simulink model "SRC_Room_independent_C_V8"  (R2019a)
settings: Solver=VariableStepAuto  StartTime=0.0  StopTime=tend  RelTol=1e-6
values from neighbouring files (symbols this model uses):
  initial_switch = zeros(10,1)    [Main_delayV8.m]
  K_amb = 1    [Main_delayV8.m]
  K_cw = -10    [Main_delayV8.m]
  K_eh = 8    [Main_delayV8.m]
  K_hw = 12    [Main_delayV8.m]
  K_rw = -5    [Main_delayV8.m]
  Kc_CW = 1/K_cw*tau_cw/(tauC2+theta_cw)    (= -0.25)    [Main_delayV8.m]
  Kc_EH = 1/K_eh*tau_eh/(tauC4+theta_eh)    (= 0.3125)    [Main_delayV8.m]
  Kc_HW = 1/K_hw*tau_hw/(tauC3+theta_hw)    (= 0.138888888889)    [Main_delayV8.m]
  Kc_RW = 1/K_rw*tau_rw/(tauC1+theta_rw)    (= -0.4)    [Main_delayV8.m]
  Tamb0 = 18    [Main_delayV8.m]
  Tamb1 = 2    [Main_delayV8.m]
  Tamb2 = 9    [Main_delayV8.m]
  Tamb3 = -5    [Main_delayV8.m]
  Tamb4 = -25    [Main_delayV8.m]
  Tamb5 = 18    [Main_delayV8.m]
  Tamb6 = 5    [Main_delayV8.m]
  tau_amb = 15    [Main_delayV8.m]
  tau_cw = 15    [Main_delayV8.m]
  tau_eh = 5    [Main_delayV8.m]
  tau_hw = 10    [Main_delayV8.m]
  tau_I_CW = min(tau_cw,4*(tauC2+theta_cw))    [Main_delayV8.m]
  tau_I_EH = min(tau_eh,4*(tauC4+theta_eh))    [Main_delayV8.m]
  tau_I_HW = min(tau_hw,4*(tauC3+theta_hw))    [Main_delayV8.m]
  tau_I_RW = min(tau_rw,4*(tauC1+theta_rw))    [Main_delayV8.m]
  tau_rw = 8    [Main_delayV8.m]
  theta_amb = 6    [Main_delayV8.m]
  theta_cw = 3    [Main_delayV8.m]
  theta_eh = 1    [Main_delayV8.m]
  theta_hw = 3    [Main_delayV8.m]
  theta_rw = 2    [Main_delayV8.m]
  Tr0 = 18    [Main_delayV8.m]
  Tsp0 = 18    [Main_delayV8.m]
  Tsp1 = 0    [Main_delayV8.m]
  Tsp2 = 0    [Main_delayV8.m]
  Tsp3 = 0    [Main_delayV8.m]
  Tsp4 = 0    [Main_delayV8.m]
  tTamb1 = tTsp1    (= 10)    [Main_delayV8.m]
  tTamb2 = 80    [Main_delayV8.m]
  tTamb3 = 140    [Main_delayV8.m]
  tTamb4 = 180    [Main_delayV8.m]
  tTamb5 = 280    [Main_delayV8.m]
  tTamb6 = 350    [Main_delayV8.m]
  tTsp1 = 10    [Main_delayV8.m]
  tTsp2 = tTsp1+40    (= 50)    [Main_delayV8.m]
  tTsp3 = tTsp2+40    (= 90)    [Main_delayV8.m]
  tTsp4 = tTsp3+40    (= 130)    [Main_delayV8.m]
  v1max = 1    [Main_delayV8.m]
  v1min = 0    [Main_delayV8.m]
  v2max = 1    [Main_delayV8.m]
  v2min = 0    [Main_delayV8.m]
  v3max = 1    [Main_delayV8.m]
  v3min = 0    [Main_delayV8.m]
  v4max = 1    [Main_delayV8.m]
  v4min = 0    [Main_delayV8.m]

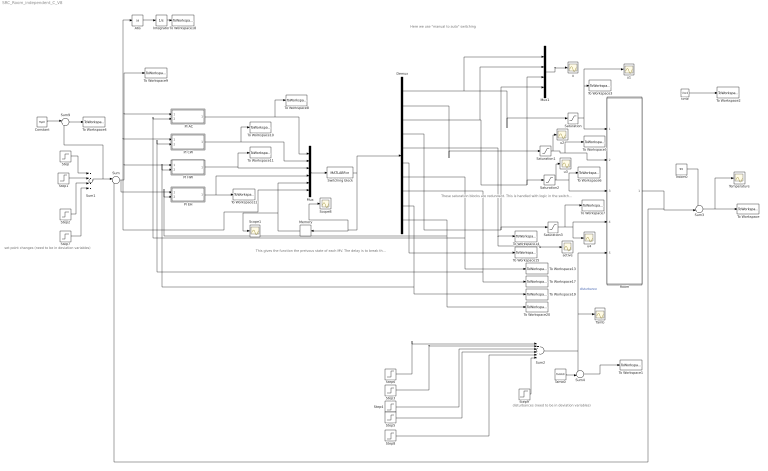
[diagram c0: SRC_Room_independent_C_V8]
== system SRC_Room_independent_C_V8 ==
  note: Here we use "manual to auto" switching
  note: disturbances (need to be in deviation variables)
  note: set point changes (need to be in deviation variables)
  note: This gives the function the preivous state of each MV. The delay is to break the algebraic loop.
  note: These saturation blocks are redundant. This is handled with logic in the switching block.
  " PI AC" : Subsystem
  Abs : Abs
  Constant : Constant  Value=Tsp0
  Demux : Demux  Outputs=10
  Integrator : Integrator
  Memory : Memory  InitialCondition=initial_switch  InheritSampleTime=on
  Mux : Mux  Inputs=6
  Mux1 : Mux
  PI CW : Subsystem
  PI EH : Subsystem
  PI HW : Subsystem
  Room : Subsystem
  Saturation : Saturate  UpperLimit=v1max  LowerLimit=v1min  ZeroCross=off
  Saturation1 : Saturate  UpperLimit=v2max  LowerLimit=v2min  ZeroCross=off
  Saturation2 : Saturate  UpperLimit=v3max  LowerLimit=v3min  ZeroCross=off
  Saturation3 : Saturate  UpperLimit=v4max  LowerLimit=v4min  ZeroCross=off
  Scope1 : Scope
  Scope8 : Scope
  Step : Step  Time=tTsp1  After=Tsp1  SampleTime=0
  Step1 : Step  Time=tTsp2  After=Tsp2  SampleTime=0
  Step2 : Step  Time=tTsp3  After=Tsp3  SampleTime=0
  Step3 : Step  Time=tTamb2  After=Tamb2  SampleTime=0
  Step4 : Step  Time=tTamb3  After=Tamb3  SampleTime=0
  Step5 : Step  Time=tTamb4  After=Tamb4  SampleTime=0
  Step6 : Step  Time=tTamb1  After=Tamb1  SampleTime=0
  Step7 : Step  Time=tTsp4  After=Tsp4  SampleTime=0
  Step8 : Step  Time=tTamb5  After=Tamb5  SampleTime=0
  Step9 : Step  Time=tTamb6  After=Tamb6  SampleTime=0
  Sum : Sum  Inputs=|+-
  Sum1 : Sum  Inputs=++++
  Sum2 : Sum  Inputs=++++++
  Sum3 : Sum  Inputs=++|
  Sum4 : Sum  Inputs=++|
  Sum9 : Sum  Inputs=|++
  Switching block : MATLABFcn  MATLABFcn=SR8  OutputDimensions=10
  Tamb : Scope
  Tamb0 : Constant  Value=Tamb0
  Temperature : Scope
  To Workspace : ToWorkspace  VariableName=T  SampleTime=-1
  To Workspace1 : ToWorkspace  VariableName=Tamb  SampleTime=-1
  To Workspace10 : ToWorkspace  VariableName=deltav2  SampleTime=-1
  To Workspace11 : ToWorkspace  VariableName=deltav3  SampleTime=-1
  To Workspace12 : ToWorkspace  VariableName=deltav4  SampleTime=-1
  To Workspace13 : ToWorkspace  VariableName=resetInt1  SampleTime=-1
  To Workspace14 : ToWorkspace  VariableName=activeMV  SampleTime=-1
  To Workspace15 : ToWorkspace  VariableName=u0active  SampleTime=-1
  To Workspace17 : ToWorkspace  VariableName=resetInt2  SampleTime=-1
  To Workspace18 : ToWorkspace  VariableName=IAE  SampleTime=-1
  To Workspace19 : ToWorkspace  VariableName=resetInt3  SampleTime=-1
  To Workspace2 : ToWorkspace  VariableName=t  SampleTime=-1
  To Workspace20 : ToWorkspace  VariableName=resetInt4  SampleTime=-1
  To Workspace3 : ToWorkspace  VariableName=u1  SampleTime=-1
  To Workspace4 : ToWorkspace  VariableName=Tsp  SampleTime=-1
  To Workspace5 : ToWorkspace  VariableName=u2  SampleTime=-1
  To Workspace6 : ToWorkspace  VariableName=u3  SampleTime=-1
  To Workspace7 : ToWorkspace  VariableName=u4  SampleTime=-1
  To Workspace8 : ToWorkspace  VariableName=deltav1  SampleTime=-1
  To Workspace9 : ToWorkspace  VariableName=T_error  SampleTime=-1
  Troom0 : Constant  Value=Tr0
  active : Scope
  time : Clock
  u{,1..4} (5 alike) : Scope
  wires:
  Room/1(T) -> Sum3/2, Sum/2  "T"
  Troom0/1 -> Sum3/1
  Sum3/1 -> Temperature/1, To Workspace/1
  Step5/1 -> Sum2/4
  Step4/1 -> Sum2/3
  Step6/1 -> Sum2/1
  Step3/1 -> Sum2/2
  Sum4/1 -> To Workspace1/1
  Tamb0/1 -> Sum4/2
  Constant/1 -> Sum9/1
  Sum1/1 -> Sum9/2, Sum/1
  Step7/1 -> Sum1/4
  Step2/1 -> Sum1/3
  Step/1 -> Sum1/1
  Step1/1 -> Sum1/2
  Sum9/1 -> To Workspace4/1
  Sum/1 -> PI EH/1(error), Mux/6, Abs/1, PI CW/1(error1), To Workspace9/1, " PI AC"/1(error), PI HW/1(error)
  Demux/1 -> Mux1/1, Saturation/1
  Demux/2 -> Saturation1/1
  Demux/3 -> Mux1/2, Mux1/3, Saturation2/1
  Demux/4 -> Saturation3/1, Mux1/4
  Saturation1/1 -> u2/1, To Workspace5/1, Room/2(vCW)
  Saturation2/1 -> u3/1, Room/3(vHW), To Workspace6/1
  Saturation3/1 -> u4/1, Room/4(vEH), To Workspace7/1
  time/1 -> To Workspace2/1
  Mux/1 -> Switching block/1
  Switching block/1 -> Scope8/1, Memory/1, Demux/1
  Demux/5 -> active/1, To Workspace14/1
  Step8/1 -> Sum2/5
  Abs/1 -> Integrator/1
  Integrator/1 -> To Workspace18/1
  Step9/1 -> Sum2/6
  Saturation/1 -> u1/1, To Workspace3/1, Room/1(vRW)
  Sum2/1 -> Sum4/1, Tamb/1, Room/5(Tamb)  "disturbance"
  " PI AC"/1(suggested u) -> Mux/1, To Workspace8/1
  PI HW/1(suggested u) -> Mux/3, To Workspace11/1
  PI EH/1(suggested u) -> To Workspace12/1, Mux/4
  Demux/6 -> To Workspace15/1
  Demux/7 -> To Workspace13/1, " PI AC"/2(reset signal)
  PI CW/1(suggested u1) -> Mux/2, To Workspace10/1
  Memory/1 -> Scope1/1, Mux/5
  Demux/8 -> To Workspace17/1, PI CW/2(reset signal)
  Demux/9 -> To Workspace19/1, PI HW/2(reset signal)
  Demux/10 -> To Workspace20/1, PI EH/2(reset signal)
  Mux1/1 -> u/1

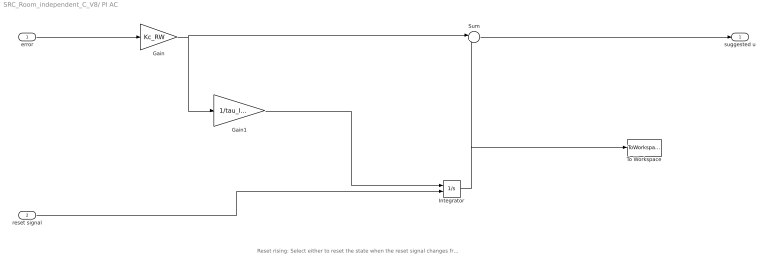
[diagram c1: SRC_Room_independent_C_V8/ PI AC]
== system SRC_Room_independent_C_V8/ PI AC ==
  note: Reset rising: Select either to reset the state when the reset signal changes from zero to a nonzero value, from a nonzero value to zero, or changes sign.
  error : Inport
  reset signal : Inport  Port=2
  Gain : Gain  Gain=Kc_RW
  Gain1 : Gain  Gain=1/tau_I_RW
  Integrator : Integrator  ExternalReset=either
  Sum : Sum  Inputs=|++
  To Workspace : ToWorkspace  VariableName=intRW  SampleTime=-1
  suggested u : Outport
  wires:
  Integrator/1 -> Sum/2, To Workspace/1
  Gain/1 -> Gain1/1, Sum/1
  Sum/1 -> suggested u/1
  error/1 -> Gain/1
  Gain1/1 -> Integrator/1
  reset signal/1 -> Integrator/2

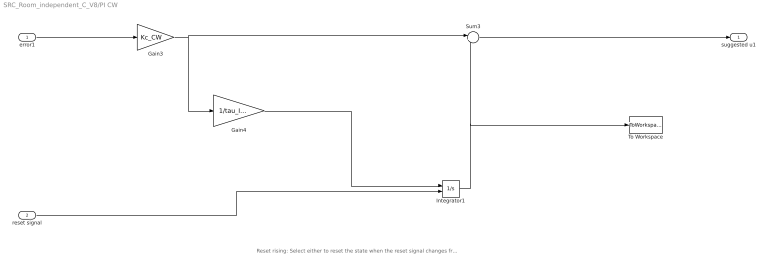
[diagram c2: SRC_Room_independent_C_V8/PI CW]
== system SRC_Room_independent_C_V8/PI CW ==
  note: Reset rising: Select either to reset the state when the reset signal changes from zero to a nonzero value, from a nonzero value to zero, or changes sign.
  error1 : Inport
  reset signal : Inport  Port=2
  Gain3 : Gain  Gain=Kc_CW
  Gain4 : Gain  Gain=1/tau_I_CW
  Integrator1 : Integrator  ExternalReset=either
  Sum3 : Sum  Inputs=|++
  To Workspace : ToWorkspace  VariableName=intCW  SampleTime=-1
  suggested u1 : Outport
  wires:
  Sum3/1 -> suggested u1/1
  error1/1 -> Gain3/1
  Gain3/1 -> Gain4/1, Sum3/1
  Integrator1/1 -> Sum3/2, To Workspace/1
  Gain4/1 -> Integrator1/1
  reset signal/1 -> Integrator1/2

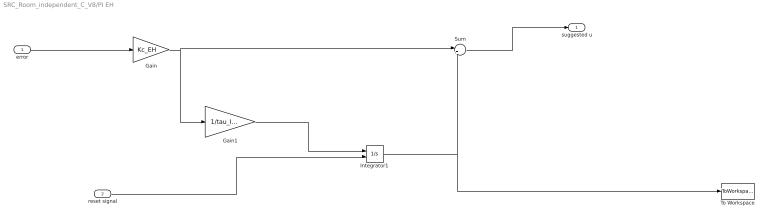
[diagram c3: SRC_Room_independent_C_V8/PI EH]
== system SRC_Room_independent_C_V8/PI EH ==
  error : Inport
  reset signal : Inport  Port=2
  Gain : Gain  Gain=Kc_EH
  Gain1 : Gain  Gain=1/tau_I_EH
  Integrator1 : Integrator  ExternalReset=either
  Sum : Sum  Inputs=|++
  To Workspace : ToWorkspace  VariableName=intEH  SampleTime=-1
  suggested u : Outport
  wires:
  Gain/1 -> Gain1/1, Sum/1
  Sum/1 -> suggested u/1
  error/1 -> Gain/1
  Gain1/1 -> Integrator1/1
  reset signal/1 -> Integrator1/2
  Integrator1/1 -> Sum/2, To Workspace/1

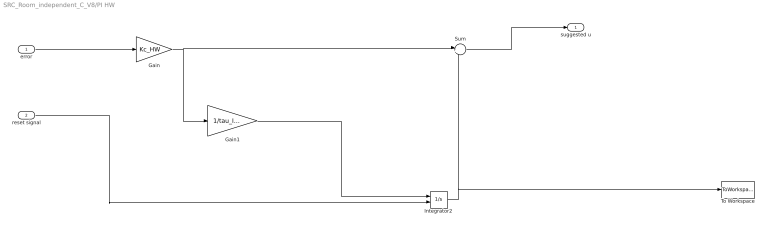
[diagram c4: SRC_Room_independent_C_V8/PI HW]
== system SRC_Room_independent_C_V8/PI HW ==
  error : Inport
  reset signal : Inport  Port=2
  Gain : Gain  Gain=Kc_HW
  Gain1 : Gain  Gain=1/tau_I_HW
  Integrator2 : Integrator  ExternalReset=either
  Sum : Sum  Inputs=|++
  To Workspace : ToWorkspace  VariableName=intHW  SampleTime=-1
  suggested u : Outport
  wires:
  Gain/1 -> Gain1/1, Sum/1
  Sum/1 -> suggested u/1
  error/1 -> Gain/1
  Gain1/1 -> Integrator2/1
  reset signal/1 -> Integrator2/2
  Integrator2/1 -> Sum/2, To Workspace/1

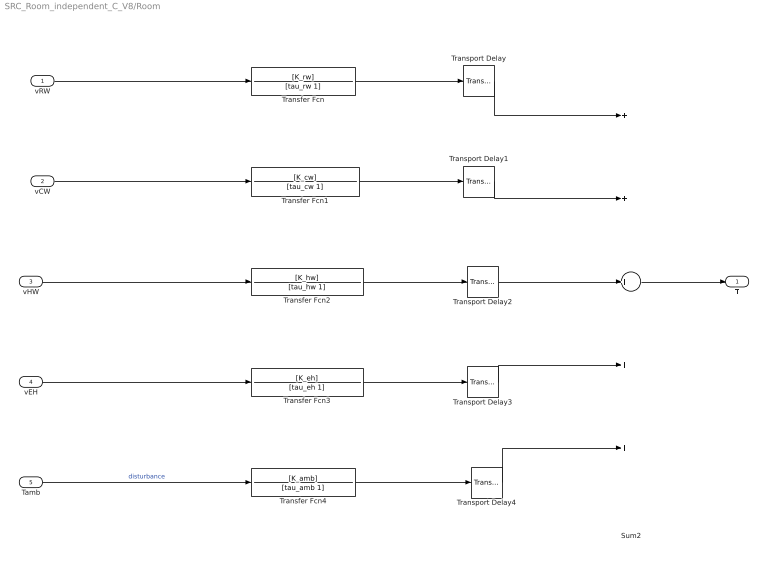
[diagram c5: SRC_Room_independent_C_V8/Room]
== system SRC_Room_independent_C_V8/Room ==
  vRW : Inport
  vCW : Inport  Port=2
  vHW : Inport  Port=3
  vEH : Inport  Port=4
  Tamb : Inport  Port=5
  Sum2 : Sum  Inputs=+++++
  Transfer Fcn : TransferFcn  Numerator=[K_rw]  Denominator=[tau_rw 1]
  Transfer Fcn1 : TransferFcn  Numerator=[K_cw]  Denominator=[tau_cw 1]
  Transfer Fcn2 : TransferFcn  Numerator=[K_hw]  Denominator=[tau_hw 1]
  Transfer Fcn3 : TransferFcn  Numerator=[K_eh]  Denominator=[tau_eh 1]
  Transfer Fcn4 : TransferFcn  Numerator=[K_amb]  Denominator=[tau_amb 1]
  Transport Delay : TransportDelay  DelayTime=theta_rw
  Transport Delay1 : TransportDelay  DelayTime=theta_cw
  Transport Delay2 : TransportDelay  DelayTime=theta_hw
  Transport Delay3 : TransportDelay  DelayTime=theta_eh
  Transport Delay4 : TransportDelay  DelayTime=theta_amb
  T : Outport
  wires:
  vRW/1 -> Transfer Fcn/1
  vCW/1 -> Transfer Fcn1/1
  vHW/1 -> Transfer Fcn2/1
  vEH/1 -> Transfer Fcn3/1
  Sum2/1 -> T/1
  Tamb/1 -> Transfer Fcn4/1  "disturbance"
  Transfer Fcn/1 -> Transport Delay/1
  Transfer Fcn1/1 -> Transport Delay1/1
  Transfer Fcn2/1 -> Transport Delay2/1
  Transfer Fcn3/1 -> Transport Delay3/1
  Transfer Fcn4/1 -> Transport Delay4/1
  Transport Delay/1 -> Sum2/1
  Transport Delay1/1 -> Sum2/2
  Transport Delay2/1 -> Sum2/3
  Transport Delay3/1 -> Sum2/4
  Transport Delay4/1 -> Sum2/5
